|Texas Instruments Incorporated
|tmux7234, 4 Data Lane 2:1 MIPI Switch (10-Channel, 2:1 Analog Switch)
[IBIS Ver]   4.1
[File name]   tmux7234.ibs
[Date]   07/09/21
[File Rev]   1.0
[Source]
| Texas Instruments Incorporated.
| ASC-INT-MPD
| 12500 TI Blvd
| Dallas, TX - 75243
[Notes]   Revision History:
| Rev 1.0: 07/09/21
| - Initial version of the model
| - Model generated from simulations in SPECTRE
| - C_comp although listed in numerical order of value are
|   obtained from varying PVT conditions. For PVT conditions for
|   each specific value refer the buffer description under
|   respective [Model]. IBIS model user is responsible for using
|   appropriate C_comp to simulate for Signal Integrity.
[Disclaimer]
| This model is designed as an aid for customers of Texas Instruments.
| TI and its licensors and suppliers make no warranties, either expressed
| or implied, with respect to this  model, including the warranties of
| merchantability or fitness for a particular purpose. The model is
| provided solely on an "as is" basis. The entire risk as to its quality
| and performance is with the customer.
| This model is subject to change without notice. Texas Instruments
| Incorporated is not responsible for updating this model.
[Copyright]
(C) Copyright 2021 Texas Instruments Incorporated.All rights reserved.
|  Component TMUX7234PW 19-pin - PW package
|  Part # TMUX7234PW
[Component]   TMUX7234PW
[Manufacturer]  TI
[Package]
|   typ   min   max
R_pkg   0.0668   NA   NA
L_pkg   2.1992nH   NA   NA
C_pkg   0.2884pF   NA   NA
[Pin]   signal_name   model_name
   1   SEL1   inbuf
   2   S1A   sterm
   3   D1   dterm
   4   S1B   sterm
   5   VSS   power
   6   GND   gnd
   7   S2B   sterm
   8   D2   dterm
   9   S2A   sterm
   10   SEL2   inbuf
   11   SEL3   inbuf
   12   S3A   sterm
   13   D3   dterm
   14   S3B   sterm
   15   ENZ   inbuf
   16   VDD   power
   17   S4B   sterm
   18   S4A   sterm
   19   SEL4   inbuf
[Series Switch Groups]
On 1 /
On 2 /
Off 1 2 /
[Series Pin Mapping]  pin_2 model_name function_table_group
|   2   3   switch_dual_5   1
|   9   8   switch_dual_5   1
|  12  13   switch_dual_5   1
|  19  18   switch_dual_5   1
|   4   3   switch_dual_5   2
|   7   8   switch_dual_5   2
|  14  13   switch_dual_5   2
|  17  18   switch_dual_5   2
   2   3   switch_dual_20   1
   9   8   switch_dual_20   1
  12  13   switch_dual_20   1
  19  18   switch_dual_20   1
   4   3   switch_dual_20   2
   7   8   switch_dual_20   2
  14  13   switch_dual_20   2
  17  18   switch_dual_20   2
|   2   3   switch_dual_15   1
|   9   8   switch_dual_15   1
|  12  13   switch_dual_15   1
|  19  18   switch_dual_15   1
|   4   3   switch_dual_15   2
|   7   8   switch_dual_15   2
|  14  13   switch_dual_15   2
|  17  18   switch_dual_15   2
|   2   3   switch_36   1
|   9   8   switch_36   1
|  12  13   switch_36   1
|  19  18   switch_36   1
|   4   3   switch_36   2
|   7   8   switch_36   2
|  14  13   switch_36   2
|  17  18   switch_36   2
|   2   3   switch_44   1
|   9   8   switch_44   1
|  12  13   switch_44   1
|  19  18   switch_44   1
|   4   3   switch_44   2
|   7   8   switch_44   2
|  14  13   switch_44   2
|  17  18   switch_44   2
|   2   3   switch_12   1
|   9   8   switch_12   1
|  12  13   switch_12   1
|  19  18   switch_12   1
|   4   3   switch_12   2
|   7   8   switch_12   2
|  14  13   switch_12   2
|  17  18   switch_12   2
|  Component TMUX7234RRQ 20-pin - RRQ package
|  Part # TMUX7234RRQ
[Component]   TMUX7234RRQ
[Manufacturer]  TI
[Package]
|   typ   min   max
R_pkg   0.067   NA   NA
L_pkg   0.937nH   NA   NA
C_pkg   0.144pF   NA   NA
[Pin]   signal_name   model_name
   1   D1   dterm
   2   S1B   sterm
   3   VSS   power
   4   GND   gnd
   5   S2B   sterm
   6   D2   dterm
   7   S2A   sterm
   8   SEL2   inbuf
   9   SEL3   inbuf
   10   S3A   sterm
   11   D3   dterm
   12   S3B   sterm
   13   VDD   power
   14   S4B   sterm
   15   D4   dterm
   16   S4A   sterm
   17   SEL4   inbuf
   18   ENZ   inbuf
   19   SEL1   inbuf
   20   S1A   sterm
[Series Switch Groups]
On 1 /
On 2 /
Off 1 2 /
[Series Pin Mapping]  pin_2 model_name function_table_group
  20   1   switch_dual_5   1
   7   6   switch_dual_5   1
  10  11   switch_dual_5   1
  16  15   switch_dual_5   1
   2   1   switch_dual_5   2
   5   6   switch_dual_5   2
  12  11   switch_dual_5   2
  14  15   switch_dual_5   2
|  20   1   switch_dual_20   1
|   7   6   switch_dual_20   1
|  10  11   switch_dual_20   1
|  16  15   switch_dual_20   1
|   2   1   switch_dual_20   2
|   5   6   switch_dual_20   2
|  12  11   switch_dual_20   2
|  14  15   switch_dual_20   2
|  20   1   switch_dual_15   1
|   7   6   switch_dual_15   1
|  10  11   switch_dual_15   1
|  16  15   switch_dual_15   1
|   2   1   switch_dual_15   2
|   5   6   switch_dual_15   2
|  12  11   switch_dual_15   2
|  14  15   switch_dual_15   2
|  20   1   switch_36   1
|   7   6   switch_36   1
|  10  11   switch_36   1
|  16  15   switch_36   1
|   2   1   switch_36   2
|   5   6   switch_36   2
|  12  11   switch_36   2
|  14  15   switch_36   2
|  20   1   switch_44   1
|   7   6   switch_44   1
|  10  11   switch_44   1
|  16  15   switch_44   1
|   2   1   switch_44   2
|   5   6   switch_44   2
|  12  11   switch_44   2
|  14  15   switch_44   2
|  20   1   switch_12   1
|   7   6   switch_12   1
|  10  11   switch_12   1
|  16  15   switch_12   1
|   2   1   switch_12   2
|   5   6   switch_12   2
|  12  11   switch_12   2
|  14  15   switch_12   2
[Model Selector] dterm
dterm_dual_5 Use for operation at +/-5V
dterm_dual_20 Use for operation at +/-20V
dterm_dual_15 Use for operation at +/-15V
dterm_36 Use for operation at 36V
dterm_44 Use for operation at 44V
dterm_12 Use for operation at 12V
[Model Selector] sterm
sterm_dual_5 Use for operation at +/-5V
sterm_dual_20 Use for operation at +/-20V
sterm_dual_15 Use for operation at +/-15V
sterm_36 Use for operation at 36V
sterm_44 Use for operation at 44V
sterm_12 Use for operation at 12V
[Model Selector] inbuf
inbuf_dual_5 Use for operation at +/-5V
inbuf_dual_20 Use for operation at +/-20V
inbuf_dual_15 Use for operation at +/-15V
inbuf_36 Use for operation at 36V
inbuf_44 Use for operation at 44V
inbuf_12 Use for operation at 12V
| switch_dual_5
[Model]   switch_dual_5
Model_type   Series_switch
|   typ   min   max
C_comp   1.008417e-11   NA   NA
[Voltage Range]   5   NA   NA
[Power Clamp Reference]   5   NA   NA
[Temperature Range]   27   NA   NA
[On]
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[Off]
|   typ   min   max
[R Series]   10G   NA   NA
| switch_dual_20
[Model]   switch_dual_20
Model_type   Series_switch
|   typ   min   max
C_comp   1.598234e-11   NA   NA
[Voltage Range]   20   NA   NA
[Power Clamp Reference]   20   NA   NA
[Temperature Range]   27   NA   NA
[On]
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[Off]
|   typ   min   max
[R Series]   10G   NA   NA
| switch_dual_15
[Model]   switch_dual_15
Model_type   Series_switch
|   typ   min   max
C_comp   1.008417e-11   NA   NA
[Voltage Range]   15   NA   NA
[Power Clamp Reference]   15   NA   NA
[Temperature Range]   27   NA   NA
[On]
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[Off]
|   typ   min   max
[R Series]   10G   NA   NA
| switch_36
[Model]   switch_36
Model_type   Series_switch
|   typ   min   max
C_comp   1.008417e-11   NA   NA
[Voltage Range]   36   NA   NA
[Power Clamp Reference]   36   NA   NA
[Temperature Range]   27   NA   NA
[On]
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[Off]
|   typ   min   max
[R Series]   10G   NA   NA
| switch_44
[Model]   switch_44
Model_type   Series_switch
|   typ   min   max
C_comp   1.598234e-11   NA   NA
[Voltage Range]   44   NA   NA
[Power Clamp Reference]   44   NA   NA
[Temperature Range]   27   NA   NA
[On]
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[Off]
|   typ   min   max
[R Series]   10G   NA   NA
| switch_12
[Model]   switch_12
Model_type   Series_switch
|   typ   min   max
C_comp   1.008417e-11   NA   NA
[Voltage Range]   12   NA   NA
[Power Clamp Reference]   12   NA   NA
[Temperature Range]   27   NA   NA
[On]
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[Off]
|   typ   min   max
[R Series]   10G   NA   NA
| Models and submodels in the file (24): dterm_dual_5 (Terminator), dterm_dual_20 (Terminator), dterm_dual_15 (Terminator), dterm_36 (Terminator), dterm_44 (Terminator), dterm_12 (Terminator), switch_dual_5 (Series_switch), switch_dual_20 (Series_switch), switch_dual_15 (Series_switch), switch_36 (Series_switch), switch_44 (Series_switch), switch_12 (Series_switch), sterm_dual_5 (Terminator), sterm_dual_20 (Terminator), sterm_dual_15 (Terminator), sterm_36 (Terminator), sterm_44 (Terminator), sterm_12 (Terminator), inbuf_dual_5 (Input), inbuf_dual_20 (Input), inbuf_dual_15 (Input), inbuf_36 (Input), inbuf_44 (Input), inbuf_12 (Input)
